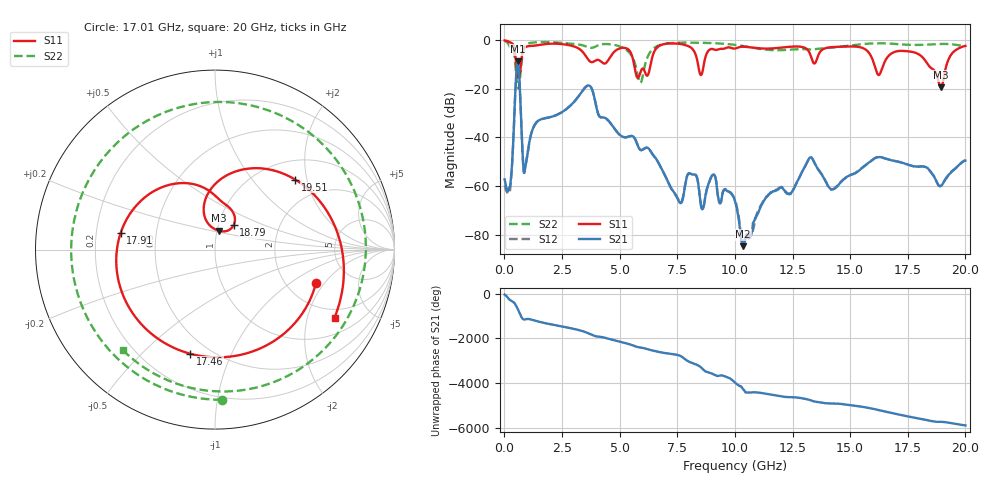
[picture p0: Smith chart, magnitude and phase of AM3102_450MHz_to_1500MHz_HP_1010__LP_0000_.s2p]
!Agilent Technologies,E8364B,MY43040894,A.07.50.67
!Agilent E8364B: A.07.50.67
!Date: Thursday, January 11, 2018 06:09:41
!Correction: S11(Full 2 Port(1,2))
!S21(Full 2 Port(1,2))
!S12(Full 2 Port(1,2))
!S22(Full 2 Port(1,2))
!S2P File: Measurements: S11, S21, S12, S22:
# Hz S  dB  R 50
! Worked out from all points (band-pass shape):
!   1601 points, 10 MHz to 20 GHz, reference 50 ohm
!   highest |S21| = -8.71 dB at 584.7 MHz (marker M1); lowest = -84.7 dB at 10.35 GHz (marker M2)
!   |S21| within 3 dB of the highest: 537 MHz to 632.7 MHz (95.7 MHz wide, 16.4 % of centre)
!   lowest |S11| = -19.4 dB at 18.94 GHz (marker M3), VSWR 1.24, Z = 51.2 + j10.8 ohm
!   |S11| at or under -10 dB: 5.627 GHz to 6.342 GHz (715.4 MHz wide, 12 % of centre); 16.05 GHz to 16.45 GHz (400.1 MHz wide, 2.46 % of centre); 18.38 GHz to 19.19 GHz (811.3 MHz wide, 4.32 % of centre)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
!   |S22| runs from -19.9 to -0.3 dB; largest |S21 - S12| = 0.00094
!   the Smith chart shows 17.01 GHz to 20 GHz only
!   S11 on the Smith chart (normalised r, x): 17.01 GHz: 2.86, -1.65; 17.46 GHz: 0.39, -0.71; 17.91 GHz: 0.31, +0.08; 18.79 GHz: 1.18, +0.33; 19.51 GHz: 1.42, +1.71; 20 GHz: 1.62, -2.97
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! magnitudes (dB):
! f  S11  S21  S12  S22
! 10 MHz  -0.1  -57.3  -59.7  -0.3
! 259.9 MHz  -0.9  -59.2  -60.6  -2.9
! 584.7 MHz  -14.7  -8.7  -8.7  -19.1
! 897.1 MHz  -3.0  -52.9  -52.7  -2.0
! 1.372 GHz  -2.1  -34.0  -34.1  -0.8
! 3.346 GHz  -4.3  -21.4  -21.4  -2.0
! 5.895 GHz  -13.4  -45.1  -45.1  -17.5
! 6.682 GHz  -2.5  -50.4  -50.4  -2.2
! 7.606 GHz  -1.5  -66.7  -66.6  -1.0
! 8.068 GHz  -2.8  -54.9  -54.8  -0.9
! 10.01 GHz  -3.4  -66.2  -65.8  -1.9
! 10.35 GHz  -2.7  -84.7  -82.4  -2.3
! 13.34 GHz  -7.8  -48.5  -48.5  -3.8
! 14.23 GHz  -2.8  -61.4  -61.4  -3.0
! 16.68 GHz  -6.3  -49.1  -49.0  -1.3
! 17.01 GHz  -4.5  -49.8  -49.9  -1.5
! 17.46 GHz  -4.5  -51.0  -51.0  -1.8
! 17.91 GHz  -5.5  -52.0  -52.0  -1.9
! 18.79 GHz  -15.3  -58.9  -59.0  -1.6
! 18.94 GHz  -19.4  -60.0  -59.8  -1.5
! 19.51 GHz  -4.5  -53.2  -53.2  -1.8
! 20 GHz  -2.3  -49.6  -49.3  -2.4
